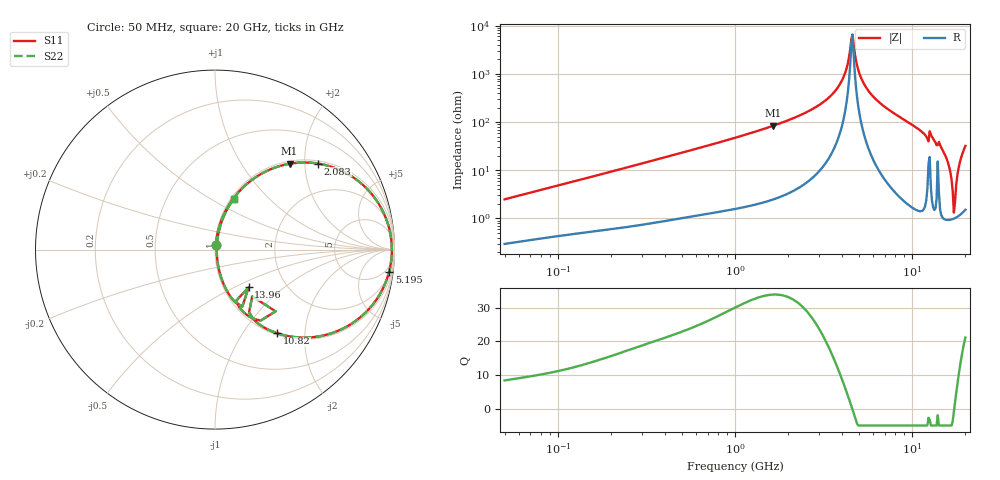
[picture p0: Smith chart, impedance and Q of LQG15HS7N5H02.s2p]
!Murata Part Number: LQG15HS7N5H02
!These Parameters are Measured in Series Mode Connection
!  o--[Z]--o
!Port1  Port2
!  o-------o
!Freq. Start=50[MHz] Stop=20[GHz], 401[Steps]
# Hz S RI R 50
!Freq.(Hz) S11(Real) S11(Imag) S21(Real) S21(Imag) S12(Real) S12(Imag) S22(Real) S22(Imag)
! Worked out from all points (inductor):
!   401 points, 50 MHz to 20 GHz, reference 50 ohm
!   read as one part in series: L = 7.8 nH near 51.52 MHz
!   highest Q = 33.9 at 1.639 GHz (marker M1), where L = 8.14 nH
!   self-resonance near 4.54 GHz
!   S11 on the Smith chart (normalised r, x): 50 MHz: 1.01, +0.05; 2.083 GHz: 1.07, +2.33; 5.195 GHz: 3, -15; 10.82 GHz: 1.03, -1.45; 13.96 GHz: 1.31, -0.60; 20 GHz: 1.03, +0.64
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5e7  0.00356 0.0246  0.9964 -0.0246  0.9964 -0.0246  0.00356 0.0246
1.364002e8  0.00908 0.0638  0.9909 -0.0638  0.9909 -0.0638  0.00908 0.0638
3.721004e8  0.0365 0.1647  0.9635 -0.1647  0.9635 -0.1647  0.0365 0.1647
1e9  0.1907 0.3766  0.8093 -0.3766  0.8093 -0.3766  0.1907 0.3766
1.639343e9  0.4154 0.4783  0.5846 -0.4783  0.5846 -0.4783  0.4154 0.4783
2.083303e9  0.5734 0.4795  0.4266 -0.4795  0.4266 -0.4795  0.5734 0.4795
2.728004e9  0.7667 0.4047  0.2333 -0.4047  0.2333 -0.4047  0.7667 0.4047
3.850025e9  0.955 0.1678  0.045 -0.1678  0.045 -0.1678  0.955 0.1678
4.212059e9  0.9777 0.0846  0.0223 -0.0846  0.0223 -0.0846  0.9777 0.0846
4.472136e9  0.9847 0.0263  0.0153 -0.0263  0.0153 -0.0263  0.9847 0.0263
4.608136e9  0.9855 -0.0034  0.0145 0.0034  0.0145 0.0034  0.9855 -0.0034
5.194772e9  0.9703 -0.1228  0.0297 0.1228  0.0297 0.1228  0.9703 -0.1228
5.944466e9  0.9174 -0.2506  0.0826 0.2506  0.0826 0.2506  0.9174 -0.2506
7.442007e9  0.7524 -0.4184  0.2476 0.4184  0.2476 0.4184  0.7524 -0.4184
1.082228e10  0.3463 -0.4659  0.6537 0.4659  0.6537 0.4659  0.3463 -0.4659
1.396067e10  0.1871 -0.2104  0.8129 0.2104  0.8129 0.2104  0.1871 -0.2104
1.573793e10  0.0354 -0.1589  0.9646 0.1589  0.9646 0.1589  0.0354 -0.1589
1.721783e10  0.0099 -0.00857  0.9901 0.00857  0.9901 0.00857  0.0099 -0.00857
1.774144e10  0.0126 0.0468  0.9874 -0.0468  0.9874 -0.0468  0.0126 0.0468
1.828096e10  0.0223 0.1045  0.9777 -0.1045  0.9777 -0.1045  0.0223 0.1045
1.88369e10  0.04 0.1637  0.96 -0.1637  0.96 -0.1637  0.04 0.1637
2e10  0.1042 0.2827  0.8958 -0.2827  0.8958 -0.2827  0.1042 0.2827
